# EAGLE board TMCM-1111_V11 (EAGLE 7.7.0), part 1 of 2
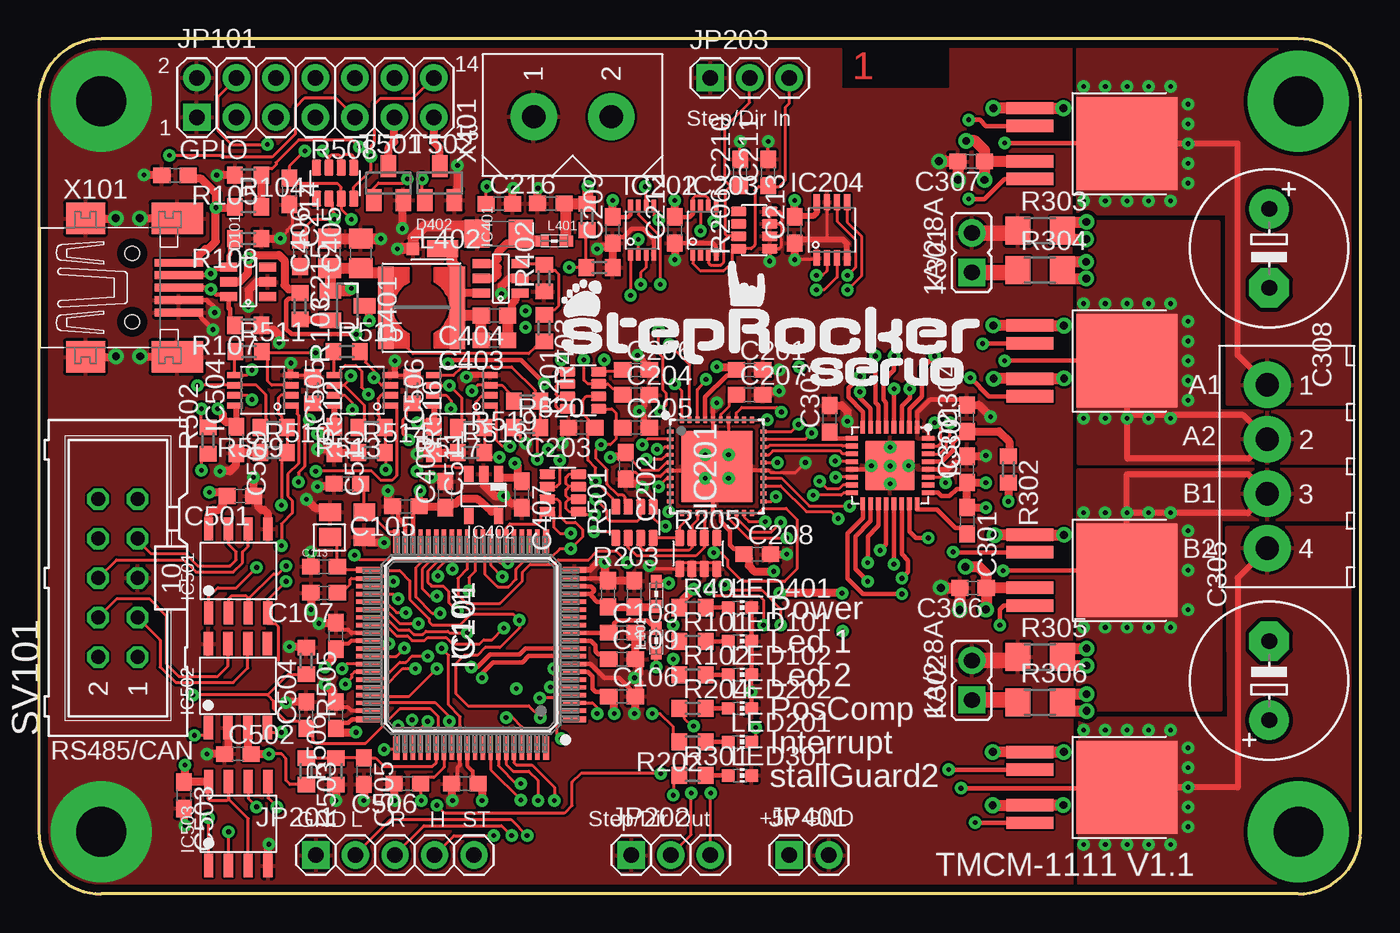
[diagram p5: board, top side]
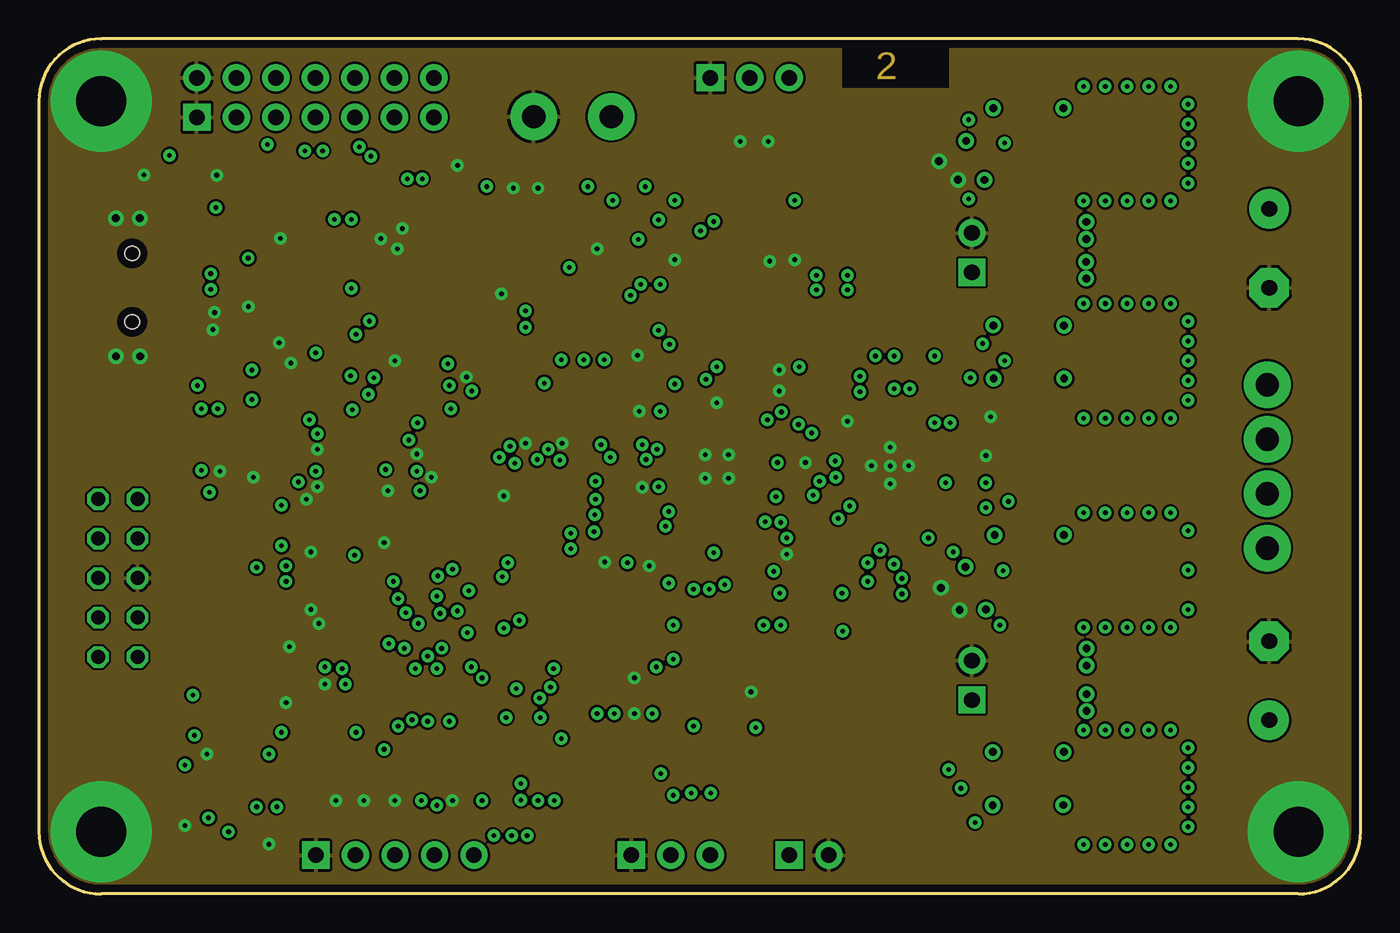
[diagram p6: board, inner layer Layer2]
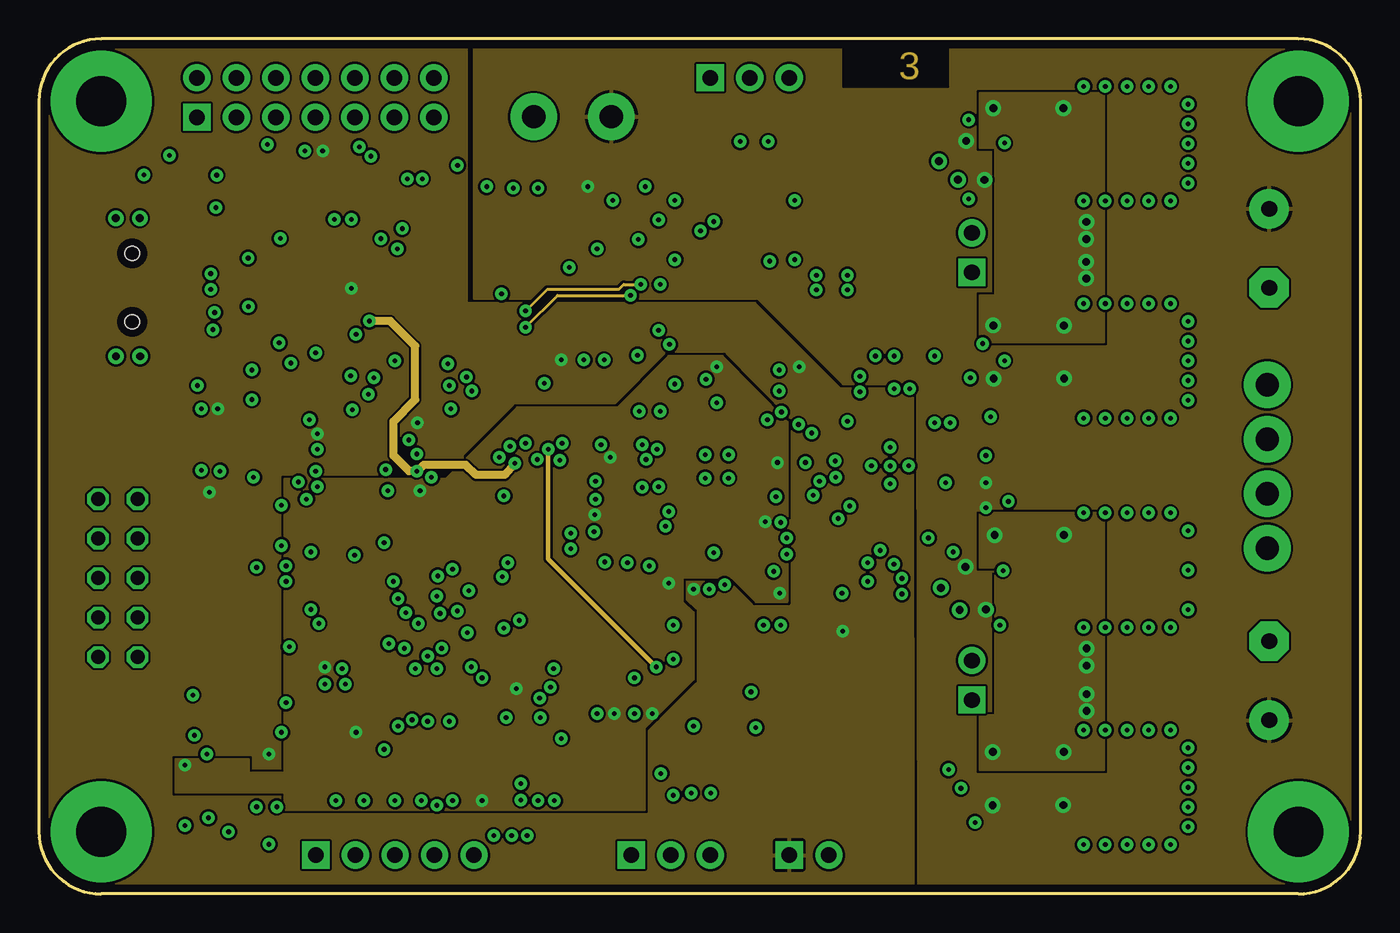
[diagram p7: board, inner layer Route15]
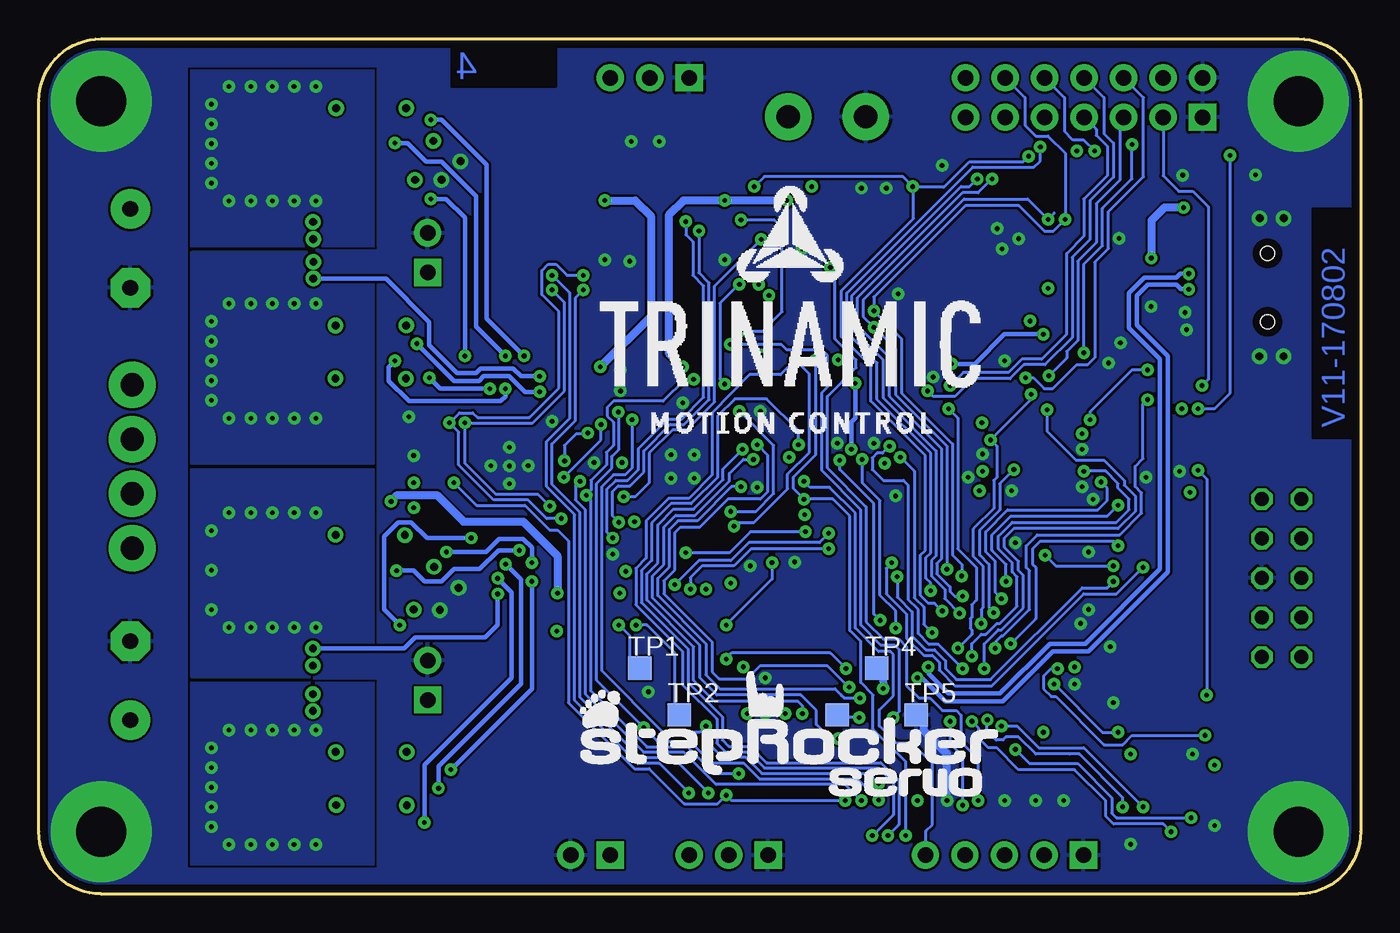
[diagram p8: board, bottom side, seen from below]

Size 85 x 55 mm. Coordinates in mm from the lower left corner, seen from the top.
Outline: 0,51 0,4 arc90 4,0 81,0 arc90 85,4 85,51 arc90 81,55 4,55 arc90 0,51
Copper layers ((1+2)*(15+16)): Top 0.035mm / dielectric 0.36mm / Layer2 0.035mm / dielectric 0.71mm / Route15 0.035mm / dielectric 0.36mm / Bottom 0.035mm
Design rules "Euro4L_1570_150": minimum track width 0.15mm, minimum drill 0.3mm, track to track 0.15mm, track to pad 0.15mm, pad to pad 0.15mm, via to via 0.15mm, smd to smd 0.15mm, copper to edge 0.5mm, drill to drill 0.3mm, minimum pad ring 0.15mm, minimum via ring 0.2mm, stop-mask expansion 0mil, vias tented up to drill 0.5mm, thermal gap 0.2mm
Net classes: 0 default: clearance 0.15 mm

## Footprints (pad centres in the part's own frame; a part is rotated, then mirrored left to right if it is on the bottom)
C0603 = smd 1.1 x 1: 1 -0.85,0; 2 0.85,0
0603 = smd 1.1 x 1: 1 -0.85,0; 2 0.85,0
E5-10,5 = drill 1.016 pad 2.54: + -2.54,0 | drill 1.016 pad 2.54 octagon: - 2.54,0
C1206 = smd 1.6 x 1.8: 1 -1.4,0; 2 1.4,0
C0805 = smd 1.3 x 1.5: 1 -0.95,0; 2 0.95,0
TMC_SOT23-6 = smd 0.6 x 1.1: 1 -0.95,-1.25; 2 0,-1.25; 3 0.95,-1.25; 4 0.95,1.25; 5 0,1.25; 6 -0.95,1.25
SOT23 = smd 1 x 1.4: 1 -0.95,-1.1; 2 0.95,-1.1; 3 0,1.1
MICRO_SMP = smd 0.8 x 0.8: A 1.25,0 | smd 2 x 1.1: C -0.65,0
LQFP80_12X12X0.5 = smd 0.4 x 1.5: 1 -4.81,-6.65; 20 4.81,-6.65; 41 4.81,6.65; 60 -4.81,6.65 | smd 0.28 x 1.5: 2 -4.25,-6.65; 3 -3.75,-6.65; 4 -3.25,-6.65; 5 -2.75,-6.65; 6 -2.25,-6.65; 7 -1.75,-6.65; 8 -1.25,-6.65; 9 -0.75,-6.65; 10 -0.25,-6.65; 11 0.25,-6.65; 12 0.75,-6.65; 13 1.25,-6.65; 14 1.75,-6.65; 15 2.25,-6.65; 16 2.75,-6.65; 17 3.25,-6.65; 18 3.75,-6.65; 19 4.25,-6.65; 42 4.25,6.65; 43 3.75,6.65; 44 3.25,6.65; 45 2.75,6.65; 46 2.25,6.65; 47 1.75,6.65; 48 1.25,6.65; 49 0.75,6.65; 50 0.25,6.65; 51 -0.25,6.65; 52 -0.75,6.65; 53 -1.25,6.65; 54 -1.75,6.65; 55 -2.25,6.65; 56 -2.75,6.65; 57 -3.25,6.65; 58 -3.75,6.65; 59 -4.25,6.65 | smd 1.5 x 0.4: 21 6.65,-4.81; 40 6.65,4.81; 61 -6.65,4.81; 80 -6.65,-4.81 | smd 1.5 x 0.28: 22 6.65,-4.25; 23 6.65,-3.75; 24 6.65,-3.25; 25 6.65,-2.75; 26 6.65,-2.25; 27 6.65,-1.75; 28 6.65,-1.25; 29 6.65,-0.75; 30 6.65,-0.25; 31 6.65,0.25; 32 6.65,0.75; 33 6.65,1.25; 34 6.65,1.75; 35 6.65,2.25; 36 6.65,2.75; 37 6.65,3.25; 38 6.65,3.75; 39 6.65,4.25; 62 -6.65,4.25; 63 -6.65,3.75; 64 -6.65,3.25; 65 -6.65,2.75; 66 -6.65,2.25; 67 -6.65,1.75; 68 -6.65,1.25; 69 -6.65,0.75; 70 -6.65,0.25; 71 -6.65,-0.25; 72 -6.65,-0.75; 73 -6.65,-1.25; 74 -6.65,-1.75; 75 -6.65,-2.25; 76 -6.65,-2.75; 77 -6.65,-3.25; 78 -6.65,-3.75; 79 -6.65,-4.25
TMC_QFN40_0.5_6.0X6.0 = smd 0.25 x 0.4: 1 -2.25,-3; 2 -1.75,-3; 3 -1.25,-3; 4 -0.75,-3; 5 -0.25,-3; 6 0.25,-3; 7 0.75,-3; 8 1.25,-3; 9 1.75,-3; 10 2.25,-3; 21 2.25,3; 22 1.75,3; 23 1.25,3; 24 0.75,3; 25 0.25,3; 26 -0.25,3; 27 -0.75,3; 28 -1.25,3; 29 -1.75,3; 30 -2.25,3 | smd 0.4 x 0.25: 11 3,-2.25; 12 3,-1.75; 13 3,-1.25; 14 3,-0.75; 15 3,-0.25; 16 3,0.25; 17 3,0.75; 18 3,1.25; 19 3,1.75; 20 3,2.25; 31 -3,2.25; 32 -3,1.75; 33 -3,1.25; 34 -3,0.75; 35 -3,0.25; 36 -3,-0.25; 37 -3,-0.75; 38 -3,-1.25; 39 -3,-1.75; 40 -3,-2.25 | smd 4.55 x 4.55: 41 0,0
US8_DCU = smd 0.3 x 0.8: 1 -0.75,-1.55; 2 -0.25,-1.55; 3 0.25,-1.55; 4 0.75,-1.55; 5 0.75,1.55; 6 0.25,1.55; 7 -0.25,1.55; 8 -0.75,1.55
SSOP08 = smd 0.4 x 1: 1 -0.975,-1.8; 2 -0.325,-1.8; 3 0.325,-1.8; 4 0.975,-1.8; 5 0.975,1.8; 6 0.325,1.8; 7 -0.325,1.8; 8 -0.975,1.8
QFN32_5X5 = smd 0.8 x 0.3: 1 -2.45,1.75; 2 -2.45,1.25; 3 -2.45,0.75; 4 -2.45,0.25; 5 -2.45,-0.25; 6 -2.45,-0.75; 7 -2.45,-1.25; 8 -2.45,-1.75; 17 2.45,-1.75; 18 2.45,-1.25; 19 2.45,-0.75; 20 2.45,-0.25; 21 2.45,0.25; 22 2.45,0.75; 23 2.45,1.25; 24 2.45,1.75 | smd 0.3 x 0.8: 9 -1.75,-2.45; 10 -1.25,-2.45; 11 -0.75,-2.45; 12 -0.25,-2.45; 13 0.25,-2.45; 14 0.75,-2.45; 15 1.25,-2.45; 16 1.75,-2.45; 25 1.75,2.45; 26 1.25,2.45; 27 0.75,2.45; 28 0.25,2.45; 29 -0.25,2.45; 30 -0.75,2.45; 31 -1.25,2.45; 32 -1.75,2.45 | smd 3.2 x 3.2: EXP 0,0
SOT23-5 = smd 0.6 x 1.05: 1 -0.95,-1.35; 2 0,-1.35; 3 0.95,-1.35; 4 0.95,1.35; 5 -0.95,1.35
SO8 = smd 1.5 x 0.6: 1 -2.7,1.905; 2 -2.7,0.635; 3 -2.7,-0.635; 4 -2.7,-1.905; 5 2.7,-1.905; 6 2.7,-0.635; 7 2.7,0.635; 8 2.7,1.905
2X07 = drill 1 pad 1.75 square: 1 -7.62,-1.27 | drill 1 pad 1.75: 2 -7.62,1.27; 3 -5.08,-1.27; 4 -5.08,1.27; 5 -2.54,-1.27; 6 -2.54,1.27; 7 0,-1.27; 8 0,1.27; 9 2.54,-1.27; 10 2.54,1.27; 11 5.08,-1.27; 12 5.08,1.27; 13 7.62,-1.27; 14 7.62,1.27
1X05 = drill 1 pad 1.75 square: 1 -5.08,0 | drill 1 pad 1.75: 2 -2.54,0; 3 0,0; 4 2.54,0; 5 5.08,0
1X03 = drill 1 pad 1.75 square: 1 -2.54,0 | drill 1 pad 1.75: 2 0,0; 3 2.54,0
1X02 = drill 1 pad 1.75 square: 1 -1.27,0 | drill 1 pad 1.75: 2 1.27,0
JP1 = drill 1 pad 1.75 square: 1 0,-1.27 | drill 1 pad 1.75: 2 0,1.27
0603' = smd 0.85 x 0.7: 1 -0.9,0; 2 0.7,0
0603'' = smd 0.85 x 0.7: 1 -0.775,0; 2 0.775,0
WE-TPC_4818/4828 = smd 1 x 5.3: 1 -2.3,0; 2 2.3,0
CHIP-LED0603 = smd 0.8 x 0.8: A 0,-0.75; C 0,0.75
R0603 = smd 1 x 1.1: 1 -0.85,0; 2 0.85,0
R_4X_1206 = smd 0.6 x 1: P$1 -1.2,-1; P$2 -0.4,-1; P$3 0.4,-1; P$4 1.2,-1; P$5 1.2,1; P$6 0.4,1; P$7 -0.4,1; P$8 -1.2,1
R1206 = smd 1.6 x 1.803: 1 -1.422,0; 2 1.422,0
ML10 = drill 0.914 octagon: 1 -5.08,-1.27; 2 -5.08,1.27; 3 -2.54,-1.27; 4 -2.54,1.27; 5 0,-1.27; 6 0,1.27; 7 2.54,-1.27; 8 2.54,1.27; 9 5.08,-1.27; 10 5.08,1.27
DUAL_DPAK_4L = smd 3 x 0.8: 1 -6.25,2.28; 2 -6.25,1.14; 4 -6.25,-1.14; 5 -6.25,-2.28 | smd 6.5 x 6: 3 0,0
TP15SQ = smd 1.5 x 1.5: TP 0,0
32005-301 = smd 3.1 x 0.5: 1 3,1.6; 2 3,0.8; 3 3,0; 4 3,-0.8; 5 3,-1.6 | smd 2.5 x 2: M1 -3,-4.45; M2 -3,4.45 | smd 3.3 x 2: M3 2.9,4.45; M4 2.9,-4.45 | hole 0.9: 0,2.2; 0,-2.2
RIACONNECT_183-04 = drill 1.5 pad 3: 1 0,5.25; 2 0,1.75; 3 0,-1.75; 4 0,-5.25
RIACONNECT_320-02 = drill 1.5 pad 3: 1 0,2.5; 2 0,-2.5
MYLIB_FA-238 = smd 1.4 x 1.15: 1 -1.1,-0.8; 2 1.1,-0.8; 3 1.1,0.8; 4 -1.1,0.8

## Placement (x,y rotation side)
C101  100nF/16V  [C0603]  8.76,46.23 180 top
C102  100nF/50V  [C0603]  27.4,7.1 180 top
C103  100nF/50V  [C0603]  19.1,11.5 90 top
C104  100nF/50V  [C0603]  19.1,16.6 90 top
C105  100nF/50V  [C0603]  23.6,24.93 180 top
C106  100nF/50V  [C0603]  37.5,12.7 0 top
C107  100nF/16V  [C0603]  18.35,19.37 180 top
C108  2µ2/16V  [C0603]  37.5,16.8 0 top
C109  2µ2/16V  [C0603]  37.5,15.1 0 top
C110  100nF/16V  [C0603]  36.6,19.3 90 top
C111  4.7µF/10V  [C0603]  38.3,19.3 90 top
C112  0603/15p/10v  [0603]  19.84,26.4 0 top
C113  0603/15p/10v  [0603]  18.34,21.05 0 top
C201  100nF  [C0603]  45.7,33.7 0 top
C202  100nF  [C0603]  37.75,27.55 270 top
C203  100nF  [C0603]  34.9,30 180 top
C204  100nF  [C0603]  38.4,32.1 0 top
C205  100nF  [C0603]  38.4,30 0 top
C206  100nF  [C0603]  38.4,33.7 0 top
C207  100nF  [C0603]  45.7,32.1 0 top
C208  100nF  [C0603]  46.2,21.85 0 top
C209  100nF  [C0603]  36.9,42.7 90 top
C210  100pF  [C0603]  45.1,46.4 90 top
C211  100pF  [C0603]  46.9,46.4 90 top
C212  100nF  [C0603]  40.9,42.7 90 top
C213  100nF  [C0603]  48.6,42.7 90 top
C214  100pF  [C0603]  16.1,45.2 270 top
C215  100pF  [C0603]  16.8,41.2 270 top
C216  100pF  [C0603]  29.6,44.4 0 top
C301  220nF 16V  [C0603]  59.69,24 270 top
C302  100nF 50V  [C0603]  59.69,27.3 90 top
C303  470nF 16V  [C0603]  50.85,30.57 90 top
C304  100nF 50V  [C0603]  59.69,30.61 90 top
C305  220µF 50V  [E5-10,5]  79.12,13.72 90 top
C306  100nF 50V  [C0603]  60.07,19.68 180 top
C307  100nF 50V  [C0603]  59.94,47.12 180 top
C308  220µF 50V  [E5-10,5]  79.12,41.53 270 top
C401  100nF/50V  [C0603]  32.93,44.41 180 top
C402  2.2µF/50V/1206  [C1206]  29.59,42.47 180 top
C403  100nF/16V  [C0603]  29.3,35.6 180 top
C404  100nF/16V  [C0603]  29.3,37.2 180 top
C405  22uF/6V3  [C0805]  20.7,41.2 90 top
C406  22uF/6V3  [C0805]  18.7,41.2 90 top
C407  4.7µF/10V  [C0603]  31.06,25.69 270 top
C408  4.7µF/10V  [C0603]  26.13,25.69 90 top
C501  100nF/50V  [C0603]  12.95,25.6 180 top
C502  100nF/50V  [C0603]  12.8,9 0 top
C503  100nF/50V  [C0603]  9.32,6.35 270 top
C504  100nF/16V  [C0603]  17.2,11.5 90 top
C505  100nF/16V  [C0603]  20.9,7.9 270 top
C506  100nF/16V  [C0603]  23.7,7.1 180 top
C509  100nF/16V  [C0603]  12.7,29.2 270 top
C510  100nF/16V  [C0603]  19,29.2 270 top
C511  100nF/16V  [C0603]  25.4,29.2 270 top
D101  SRV05-4  [TMC_SOT23-6]  13.46,39.37 90 top
D401  PMEG2005CT  [SOT23]  19.85,37.84 270 top
D402  MSS1P6  [MICRO_SMP]  25.3,41.5 180 top
DRILEGEND  [DRILEGEND]  not placed on the board
IC101  MK20DX128VLK7  [LQFP80_12X12X0.5]  27.8,16.04 90 top
IC201  TMC4361-LA  [TMC_QFN40_0.5_6.0X6.0]  43.6,27.5 270 top
IC202  SN74LVC3G17DCUR  [US8_DCU]  38.8,42.7 0 top
IC203  SN74LVC3G17DCUR  [US8_DCU]  42.8,42.7 0 top
IC204  74AHCT2G125DP  [SSOP08]  51,42.7 0 top
IC301  TMC262-LA  [QFN32_5X5]  54.74,27.56 270 top
IC401  LM2841YMK  [TMC_SOT23-6]  29.7,39.6 90 top
IC402  LP2985AIM5-3.3  [SOT23-5]  28.61,25.67 180 top
IC501  SN65HVD3082ED  [SO8]  12.83,20.77 90 top
IC502  TJA1050T  [SO8]  12.8,13.4 90 top
IC503  AT25128B  [SO8]  12.83,4.52 90 top
IC504  74AHCT2G125DP  [SSOP08]  14.4,32.4 90 top
IC505  74AHCT2G125DP  [SSOP08]  20.8,32.4 90 top
IC506  74AHCT2G125DP  [SSOP08]  27.2,32.4 90 top
JP101  nv  [2X07]  17.78,51.23 0 top
JP201  nv  [1X05]  22.9,2.5 0 top
JP202  nv  [1X03]  40.64,2.5 0 top
JP203  nv  [1X03]  45.72,52.5 0 top
JP401  [1X02]  49.53,2.5 0 top
K301  nv  [JP1]  60,41.25 0 top
K302  nv  [JP1]  60,13.75 0 top
L101  600R/100MHz  [0603']  39.7,19.2 270 top
L102  600R/100MHz  [0603']  39.7,16.2 270 top
L401  600R@100MHz/1A  [0603'']  33.14,42 180 top
L402  WE-TPC_33UH/0.5A  [WE-TPC_4818/4828]  24.6,37.7 180 top
LED101  yellow  [CHIP-LED0603]  45.09,16.26 270 top
LED102  yellow  [CHIP-LED0603]  45.09,14.1 270 top
LED201  orange  [CHIP-LED0603]  45.09,9.78 270 top
LED202  yellow  [CHIP-LED0603]  45.09,11.94 270 top
LED301  red  [CHIP-LED0603]  45.09,7.62 270 top
LED401  orange  [CHIP-LED0603]  45.09,18.41 270 top
R101  680R  [R0603]  42.04,16.26 0 top
R102  680R  [R0603]  42.04,14.1 0 top
R103  0R  [R0603]  16.8,37.8 270 top
R104  10K  [R0603]  13.46,44.2 0 top
R105  43K n.b.  [R0603]  13.46,46.23 180 top
R107  470k  [R0603]  13.46,36.58 180 top
R108  470k  [R0603]  13.46,42.16 180 top
R201  4k7  [R_4X_1206]  35,32.4 90 top
R202  1K8  [R0603]  42.04,9.78 180 top
R203  4k7  [R_4X_1206]  38.3,23.9 180 top
R204  1K8  [R0603]  42.04,11.94 0 top
R205  12K  [R_4X_1206]  42.4,21.9 0 top
R206  4k7  [R_4X_1206]  46,42.7 90 top
R301  1K8  [R0603]  42.04,7.62 0 top
R302  0R  [R0603]  62.36,27.3 270 top
R303  0R220  [R1206]  64.39,42.67 0 top
R304  0R1  [R1206]  64.39,40.13 0 top
R305  0R220  [R1206]  64.39,15.24 0 top
R306  0R1  [R1206]  64.39,12.32 0 top
R401  1K8  [R0603]  42.04,18.41 0 top
R402  4k87  [R0603]  32.5,39.6 90 top
R403  27k  [R0603]  32.5,36.4 270 top
R501  4k7  [R_4X_1206]  33.7,25.8 270 top
R502  22k  [R0603]  10.88,29.17 90 top
R503  5k6  [R0603]  17.2,7.9 270 top
R504  82k  [R0603]  35.25,43.55 90 top
R505  10k  [R0603]  17.2,15 270 top
R506  10k  [R0603]  19.1,7.9 90 top
R507  10k  [R0603]  36.05,40.3 180 top
R508  1k8  [R_4X_1206]  19.05,45.72 0 top
R509  1k  [R0603]  15.1,30 180 top
R510  1M n.b.  [R0603]  15.1,28.4 0 top
R511  1k  [R0603]  13.5,34.9 0 top
R512  1M n.b.  [R0603]  17.6,32.4 270 top
R513  1k  [R0603]  21.4,30 180 top
R514  1M n.b.  [R0603]  21.4,28.4 0 top
R515  1k  [R0603]  19.8,34.9 0 top
R516  1M n.b.  [R0603]  24,32.4 270 top
R517  1k  [R0603]  27.8,30 180 top
R518  1M n.b.  [R0603]  27.8,28.4 0 top
R519  1k  [R0603]  31.4,31.7 180 top
R520  1M n.b.  [R0603]  31.4,30 0 top
SV101  nv  [ML10]  5.08,20.32 90 top
T301  FDD8424H  [DUAL_DPAK_4L]  69.98,48.26 0 top
T302  FDD8424H  [DUAL_DPAK_4L]  69.98,34.29 0 top
T303  FDD8424H  [DUAL_DPAK_4L]  69.98,20.83 0 top
T304  FDD8424H  [DUAL_DPAK_4L]  69.98,6.86 0 top
T501  BSS138  [SOT23]  22.48,45.72 0 top
T502  BSS138  [SOT23]  25.78,45.72 0 top
TP1  TPTP15SQ  [TP15SQ]  46.35,14.52 0 bottom
TP2  TPTP15SQ  [TP15SQ]  43.81,11.52 0 bottom
TP3  TPTP15SQ  [TP15SQ]  33.66,11.52 0 bottom
TP4  TPTP15SQ  [TP15SQ]  31.11,14.52 0 bottom
TP5  TPTP15SQ  [TP15SQ]  28.57,11.52 0 bottom
X101  MINI-USB-SCHIELD-32005-301  [32005-301]  6,39 0 top
X301  RIACONNECT_183-04  [RIACONNECT_183-04]  79,27.5 0 top
X401  TMC_POWER_CONNECTOR  [RIACONNECT_320-02]  34.32,50 90 top
Y101  16MHZ-3.2X2.5  [MYLIB_FA-238]  19.83,23.75 0 top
